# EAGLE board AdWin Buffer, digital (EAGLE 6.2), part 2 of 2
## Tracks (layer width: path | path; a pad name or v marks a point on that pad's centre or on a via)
+5V  (via drill 0.71)
  Top 0.406: IC3.21 301.75,53.75 301,53 301,49.25 299.5,47.75 298.5,47.75 C20.2 298.25,47.5 298,47.5 296.12,45.62 | 295.75,39.25 300.5,39.25 302.25,37.5 302.25,37 IC11.21 | 295.75,39.25 292,39.25 289.75,37 IC11.16 | 296.12,45.62 295.75,45.25 295.75,39.25 | 249.12,62.88 248.5,62.25 IC2.16 | 249.12,62.88 249.25,63 249.25,63.75 C4.2 | IC7.16 248.5,43 248.75,43.25 248.75,45.5 C18.2 249,45.75 249,46.75 250.12,47.88 | 250.62,61.38 250.75,61.25 250.75,48.5 250.12,47.88 | 250.62,61.38 249.12,62.88 | IC9.16 270.5,43.25 271.75,44.5 271.75,45.5 C16.2 271.75,45.75 271.75,47.5 | C5.2 271,64.5 271,62.25 270.75,62 IC1.16 | C3.2 287.5,65 287.5,66 286,67.5 283.25,67.5 282.25,66.5 273.75,66.5 272,64.75 271.38,64.75 C5.2 | 271.25,64.5 C5.2 | IC3.16 288.75,53.75 288.75,52.5 287.75,51.5 279.75,51.5 279.5,51.75 279.5,52.25 278.25,53.5 276.75,53.5 275.25,55 275.25,56.5 273.75,58 273.75,60.75 272.25,62.25 270.66,62.25 IC1.16 | 271.75,47.5 271.75,49.5 267.75,53.5 267.75,60.75 267.88,60.88 | 267.88,60.88 269.25,62.25 270.5,62.25 IC1.16 | 267.88,60.88 263.75,65 257.5,65 254,61.5 250.75,61.5 250.62,61.38 | 296.12,45.62 294.25,47.5 271.75,47.5 | F2.1A 182,59.75 172.5,69.25 167.75,69.25 C6.2 167.5,69.25 164,69.25 ZD1.2 163.75,69.25 163.25,68.75 161,68.75 159.48,67.23 147.51,67.23 143.25,62.75 142,62.75 141.75,63 120.75,63 v120.5,62.75 | C21.2 72.5,19.75 76.75,19.75 85.5,28.5 85.5,33.5 IC10.16 85.75,33.75 87,33.75 88,34.75 88,49.25 87.5,49.75 87.5,52 87.62,52.12 | 107.88,32.38 109,33.5 IC8.16 | 107.88,32.38 107,31.5 104.75,31.5 C19.2 | 104.75,40.75 104.75,35.5 107.88,32.38 | 104.75,40.75 104.75,41.25 C17.2
  Top 0.406: 104.75,40.75 106.5,42.5 v106.5,47.5 106.5,50 107.75,51.25 108.5,51.25 C10.2 108.75,51.5 108.75,53.25 109,53.5 IC4.16 109.25,53.25 v111,53.25 | 67.25,61.75 67.25,61 IC6.16 67.25,62 | IC6.21 54.75,61 61,67.25 61.5,67.25 C11.2 61.75,67.25 61.75,66.5 62.5,65.75 62.5,63.75 63.25,63 65.75,63 66.75,62 67.25,62 | 79.75,51.25 75.75,51.25 68.88,44.38 | 79.75,51.25 84.5,51.25 C9.2 84.75,51.5 84.75,52.5 85.5,53.25 IC5.16 85.75,53.25 86.5,53.25 87.62,52.12 | 68.88,44.38 67.5,43 67.5,42 IC12.16 | IC12.21 54.75,42 57.25,44.5 68.75,44.5 68.88,44.38 | 67.25,62 68.25,63 72.75,63 73.5,62.25 73.5,59.5 76,57 79,57 79.75,56.25 79.75,51.25 | 87.62,52.12 v92.25,47.5 | v243.75,50.25 244,50 248,50 250.12,47.88
  Bottom 0.406: v92.25,47.5 v106.5,47.5 | v111,53.25 v120.5,62.75 | F2.1A 182.25,59.5 216.25,59.5 222.5,53.25 240.75,53.25 v243.75,50.25
AGND  (via drill 0.71)
  other vias: 82.5,52.75 86.5,47.25 86.25,51.5 83.75,44.5 82.25,39 268.25,65.75 291.75,66.5 304,49 268.25,34.25 273.75,46 113.5,30.25 113.5,36.25 113.5,33.25 61.75,69 68.75,30.75 269,46 269,50.75 273.75,50.75 285.75,66.25 268.75,60.25 300.75,66.75 303.75,67
  pour Top (isolate 0.203): 0,96.52 0,5.08 169.03,5.08 169.03,0 330.2,0 330.2,96.52 171.45,96.52 171.45,88.9 164.47,88.9 164.47,92.08 158.12,92.08 158.12,96.52
  pour Bottom (isolate 0.203): 0,96.52 0,0 330.2,0 330.2,96.52
D0  (via drill 0.51)
  Top 0.178: v161.75,71 v165.25,71 | v139.75,55 138.5,53.75 138.5,49.75 J1.19 | IC2.3 239.25,59.75 239,59.5 237,59.5 236.75,59.25 v236.5,59.25
  Bottom 0.178: v165.25,71 170.75,65.5 222,65.5 228.25,59.25 v236.5,59.25 | v161.75,71 157.75,67 141.25,67 140,65.75 140,55.25 v139.75,55
D1  (via drill 0.51)
  Top 0.178: v156.75,64.5 167.75,64.5 176,56.25 226,56.25 235,65.25 240,65.25 243,62.25 243,60 241.5,58.5 239.5,58.5 IC2.4 | v139.75,53.75 139.75,47 J1.37
  Bottom 0.178: v156.75,64.5 156.25,64.5 154.25,66.5 141.5,66.5 140.5,65.5 140.5,54.5 v139.75,53.75
D2  (via drill 0.51)
  Top 0.178: v237.25,57.25 239.25,57.25 IC2.5 | v141,53.75 141,49.75 J1.18
  Bottom 0.178: v237.25,57.25 228.75,57.25 222.5,63.5 174.5,63.5 170.25,59.25 170.25,56.75 169.5,56 161.5,56 156.25,61.25 156.25,63.75 154,66 141.75,66 141,65.25 v141,53.75
D3  (via drill 0.51)
  Top 0.178: v237.25,56 239.25,56 IC2.6 | v165,53.25 162,53.25 159,50.25 159,49 158.25,48.25 154.5,48.25 153.5,49.25 153.5,50.25 152.25,51.5 146.5,51.5 145.25,50.25 145.25,49.25 143,47 142.5,47 J1.36
  Bottom 0.178: v237.25,56 229.25,56 222.25,63 174.75,63 170.75,59 170.75,56.62 168.5,54.38 166.25,54.38 165.12,53.25 v165,53.25
D4  (via drill 0.51)
  Top 0.178: v259.5,59.75 261.25,59.75 IC1.3 | v168.25,75 153.75,75 v143.5,64.75 | v143.25,56 143.25,50.25 143.75,49.75 J1.17
  Bottom 0.178: v259.5,59.75 248.25,59.75 240,68 181.25,68 174.25,75 v168.25,75 | v143.5,64.75 142.5,64.75 142,64.25 142,57.25 v143.25,56
D5  (via drill 0.51)
  Top 0.178: v263.25,58.5 261.5,58.5 IC1.4 | v163,63.75 156,63.75 v155.5,63.25
  Bottom 0.178: v263.25,58.5 262.75,58.5 260,55.75 250,55.75 247.5,58.25 228.5,58.25 222.75,64 163.25,64 v163,63.75 | v155.5,63.25 146.75,63.25 144.5,65.5 142,65.5 141.5,65 141.5,56.5 144.5,53.5 147.5,53.5 150.75,50.25 150.75,49.25 149.75,48.25 147,48.25 145.75,47 145.25,47 J1.35
D6  (via drill 0.51)
  Top 0.178: v259.5,57.75 260,57.25 261.25,57.25 IC1.5 | v177,67.5 168.75,75.75 v156.25,75.75 | v139,56.5 139.5,56.5 142.5,53.5 v142.5,52.25
  Bottom 0.178: v259.5,57.75 249.5,57.75 239.75,67.5 v177,67.5 | v156.25,75.75 148,67.5 141,67.5 139.5,66 139.5,57.25 139,56.75 v139,56.5 | v142.5,52.25 143.75,52.25 146.5,49.5 J1.16
D7  (via drill 0.51)
  Top 0.178: v259.5,56.5 260,56 261.25,56 IC1.6 | v230.5,65.25 182.75,65.25 169.5,78.5 150.25,78.5 v141,69.25 | v136.25,56.5 136.25,48 138.75,45.5 147,45.5 148.25,46.75 J1.34
  Bottom 0.178: v259.5,56.5 250,56.5 241.25,65.25 v230.5,65.25 | v141,69.25 138.25,66.5 138.25,58.5 v136.25,56.5
D8  (via drill 0.51)
  Top 0.178: v93,56 94.5,56 IC5.3
  Bottom 0.178: v93,56 97.75,51.25 128.5,51.25 130.25,53 145.75,53 149.25,49.5 J1.15
D9  (via drill 0.51)
  Top 0.178: v93,57.25 94.5,57.25 IC5.4
  Bottom 0.178: v93,57.25 92.25,56.5 92.25,55.5 97,50.75 122.5,50.75 129.5,43.75 148,43.75 151,46.75 J1.33
D10  (via drill 0.51)
  Top 0.178: v91.75,57.25 92.75,58.25 94.5,58.25 IC5.5 | J1.14 152.25,49.5 152.25,46.25 149.25,43.25 128.5,43.25 127.75,44 v127.75,44.25
  Bottom 0.178: v91.75,57.25 91.75,55.25 96.75,50.25 121.75,50.25 v127.75,44.25
D11  (via drill 0.51)
  Top 0.178: v91,55.25 91,57.75 92.75,59.5 94.5,59.5 IC5.6
  Bottom 0.178: v91,55.25 96.5,49.75 121,49.75 127.5,43.25 150.25,43.25 153.75,46.75 J1.32
D12  (via drill 0.51)
  Top 0.178: v116.5,56 118,56 IC4.3 | v125.5,57.25 147.25,57.25 154.75,49.75 J1.13
  Bottom 0.178: v116.5,56 124.25,56 v125.5,57.25
D13  (via drill 0.51)
  Top 0.178: v116.5,57.25 118,57.25 IC4.4 | v124.25,57.25 125,58 v145.75,58
  Bottom 0.178: v124.25,57.25 v116.5,57.25 | v145.75,58 153.5,50.25 153.5,49.25 155.75,47 156.25,47 J1.31
D14  (via drill 0.51)
  Top 0.178: v116,59.5 117,58.5 118,58.5 IC4.5 | v133.75,59 148,59 157.5,49.5 J1.12
  Bottom 0.178: v116,59.5 120.25,63.75 131,63.75 133.75,61 v133.75,59
D15  (via drill 0.51)
  Top 0.178: v142.75,63.75 118,63.75 116.5,62.25 116.5,60.25 117,59.75 118,59.75 IC4.6
  Bottom 0.178: v142.75,63.75 156.25,50.25 156.25,49.25 158.5,47 159,47 J1.30
D16  (via drill 0.51)
  Top 0.178: v255,39 255.25,38.75 262.75,38.75 263,39 263,39.75 262.25,40.5 261.5,40.5 IC9.3 | v246.5,31 179,31 165.25,44.75 162.75,44.75 v162.5,45
  Bottom 0.178: v255,39 254.5,39 v246.5,31 | v162.5,45 161.75,45 160.5,46.25 160.5,49.5 J1.11
D17  (via drill 0.51)
  Top 0.178: v167.5,48.5 168.75,47.25 168.75,46.25 182.75,32.25 241.75,32.25 244.5,35 244.5,38.5 247.25,41.25 259.5,41.25 259.75,41 259.75,40 260.25,39.5 261.25,39.5 IC9.4
  Bottom 0.178: v167.5,48.5 166.75,48.5 166.5,48.25 163.5,48.25 162,46.75 J1.29
D18  (via drill 0.51)
  Top 0.178: v166.75,53 163.25,49.5 J1.10 | IC9.5 261.34,38.25 254.5,38.25 253,39.75 v250.25,39.75
  Bottom 0.178: v250.25,39.75 246.25,39.75 244.25,41.75 218.25,41.75 212.25,47.75 212.25,51 210.25,53 v166.75,53
D19  (via drill 0.51)
  Top 0.178: v253.75,36.75 261.25,36.75 IC9.6 | v248.75,31.75 179.25,31.75 164.75,46.25 164.75,46.75 J1.28
  Bottom 0.178: v248.75,31.75 v253.75,36.75
D20  (via drill 0.51)
  Top 0.178: v241,40.5 239.5,40.5 IC7.3 | v176.25,36 166,46.25 166,49.5 J1.9
  Bottom 0.178: v241,40.5 241.75,39.75 241.75,36.25 241.5,36 v176.25,36
D21  (via drill 0.51)
  Top 0.178: v241,39.25 239.5,39.25 IC7.4 | v174.5,39.25 167.5,46.25 167.5,46.75 J1.27
  Bottom 0.178: v174.5,39.25 v241,39.25
D22  (via drill 0.51)
  Top 0.178: v241,38 239.5,38 IC7.5 | v179.75,38 171.5,46.25 171.5,47.25 169.25,49.5 168.75,49.5 J1.8
  Bottom 0.178: v179.75,38 v241,38
D23  (via drill 0.51)
  Top 0.178: v241,36.75 239.5,36.75 IC7.6 | v179.75,36.75 170.25,46.25 170.25,46.75 J1.26
  Bottom 0.178: v179.75,36.75 v241,36.75
D24  (via drill 0.51)
  Top 0.178: v93,36.25 94.5,36.25 IC10.3 | J1.7 171.25,49.5 169.25,51.5 166,51.5 164.5,50 164.5,49 163.75,48.25 161.25,48.25 160.5,47.5 160.5,46.5 156,42 126,42 124.5,43.5 v123.5,43.5
  Bottom 0.178: v93,36.25 98.25,36.25 104.75,42.75 122.75,42.75 v123.5,43.5
D25  (via drill 0.51)
  Top 0.178: v93,37.5 94.5,37.5 IC10.4 | v123.5,42.25 v122.25,43.5
  Bottom 0.178: v93,37.5 98.75,37.5 104.75,43.5 v122.25,43.5 | v123.5,42.25 163.25,42.25 166.5,45.5 171.25,45.5 172.75,47 J1.25
D26  (via drill 0.51)
  Top 0.178: v93,38.75 94.5,38.75 IC10.5 | v155,59.75 154.75,59.75 154.5,59.5 134.75,59.5 134.25,60 131.25,60 129.75,58.5 124.25,58.5 123.25,57.5 123.25,49.5 121.25,47.5 v121.25,47.25
  Bottom 0.178: v93,38.75 99.25,38.75 105.75,45.25 119.25,45.25 v121.25,47.25 | v155,59.75 163.25,51.5 172.25,51.5 174.25,49.5 J1.6
D27  (via drill 0.51)
  Top 0.178: v93,40 94.5,40 IC10.6 | v101.25,42 103.75,39.5 v103.75,39.25 | v176.25,42.75 176.25,46.25 175.75,46.75 J1.24
  Bottom 0.178: v93,40 99.25,40 v101.25,42 | v103.75,39.25 114.25,39.25 129.75,23.75 132.5,23.75 133.5,24.75 133.5,26.5 143.25,36.25 169.75,36.25 v176.25,42.75
D28  (via drill 0.51)
  Top 0.178: v117.75,44.5 116.5,43.25 116.5,36.75 117,36.25 118,36.25 IC8.3 | J1.5 176.75,49.5 171.25,55 161,55 155.5,60.5 154.25,60.5 153.75,60 137.5,60 v137,60.5 | v121,44.5 126.5,50 126.5,51.5 131.5,56.5 v133,56.5
  Bottom 0.178: v121,44.5 v117.75,44.5 | v137,60.5 v133,56.5
D29  (via drill 0.51)
  Top 0.178: v120,37.5 118.25,37.5 IC8.4
  Bottom 0.178: v120,37.5 160,37.5 167,44.5 176.25,44.5 178.5,46.75 J1.23
D30  (via drill 0.51)
  Top 0.178: v120,38.75 118.25,38.75 IC8.5
  Bottom 0.178: v120,38.75 160.5,38.75 166.75,45 175.75,45 177,46.25 177,47.25 179.25,49.5 179.75,49.5 J1.4
D31  (via drill 0.51)
  Top 0.178: v120,40 IC8.6 | v178.25,43.5 181,46.25 181,46.75 J1.22
  Bottom 0.178: v120,40 119.25,39.25 119.25,37 119.5,36.75 169,36.75 175.75,43.5 v178.25,43.5
N$1  (via drill 0.51)
  Top 0.178: v245.5,53 245.5,58 247,59.5 248.25,59.5 IC2.14 | v302,48.75 306.5,53.25 306.5,53.75 IC3.23
  Bottom 0.178: v245.5,53 249.75,48.75 v302,48.75
N$2  (via drill 0.51)
  Top 0.178: v246.75,53 246,53.75 246,57.25 247,58.25 248.25,58.25 IC2.13 | v302,50.25 304.25,52.5 304.25,53.75 IC3.22
  Bottom 0.178: v246.75,53 250.5,49.25 301,49.25 v302,50.25
N$3  (via drill 0.51)
  Top 0.178: v249.75,52.25 250.25,52.75 250.25,56.5 249.75,57 248.5,57 IC2.12
  Bottom 0.178: v249.75,52.25 273.5,52.25 276,49.75 295,49.75 299,53.75 IC3.20
N$4  (via drill 0.51)
  Top 0.178: v246.75,55.75 248.25,55.75 IC2.11
  Bottom 0.178: v246.75,55.75 249.25,55.75 249.75,55.25 271.25,55.25 276.25,50.25 293,50.25 296.5,53.75 IC3.19
N$5  (via drill 0.51)
  Top 0.178: v70.75,68 70,68.75 69.5,68.75 59.5,78.75 v59.5,79.25 | IC5.14 82.62,55.88 v77.25,61.25
  Bottom 0.178: v70.75,68 77.25,61.5 v77.25,61.25 | v59.5,79.25 51.5,79.25 49.25,77 49.25,61.25 49.5,61 IC6.23
N$6
  Top 0.178: IC5.13 85.75,57.25 86.75,57.25 88,58.5 88,63 83.75,67.25 66.25,67.25 63,70.5 60.5,70.5 52.25,62.25 52.25,61 IC6.22
N$7  (via drill 0.51)
  Top 0.178: v273.25,55.75 270.75,55.75 IC1.11
  Bottom 0.178: v273.25,55.75 276,55.75 279.5,52.25 282.25,52.25 283.75,53.75 IC3.14
N$8  (via drill 0.51)
  Top 0.178: v61.25,65.25 57,61 IC6.20 | IC5.12 85.75,58.5 86.75,58.5 87.5,59.25 87.5,62.75 84.5,65.75 65.25,65.75 64.75,65.25 v64.5,65.25
  Bottom 0.178: v61.25,65.25 v64.5,65.25
N$9  (via drill 0.51)
  Top 0.178: v66.5,64.25 77.75,64.25 82.25,59.75 85.5,59.75 IC5.11
  Bottom 0.178: v66.5,64.25 62.5,64.25 59.75,61.5 59.75,61 IC6.19
N$10  (via drill 0.51)
  Top 0.178: v286.75,56.5 281.5,56.5 281,56 v279.25,56 277.5,56 276.75,56.75 276.75,57.75 277,58 278,58 278.75,57.25 280.75,57.25 281,57.5 281,58.5 279,60.5 v279,63.5 | v295.75,66 296.5,65.25 296.5,61.75 IC3.6 | v279,68.5 287,68.5 v287.5,68
  Bottom 0.178: v279.25,56 280,56.75 283.25,56.75 R1.4A | v286.75,56.5 287.5,56.5 287.75,56.75 288.75,56.75 R2.4A | v295.75,66 294.5,66 292.5,68 v287.5,68 | v279,63.5 v279,68.5
N$11  (via drill 0.51)
  Top 0.178: v279.75,61 282.25,58.5 287.5,58.5 288,58 v293.5,58 | v288.25,56 v292.5,56 | v293,60 293.25,59.75 294.25,59.75 295,60.5 295,66.5 295.25,66.75 297.5,66.75 301.5,62.75 301.5,61.75 IC3.4
  Bottom 0.178: v279.75,61 278.25,59.5 278.25,55.75 278.75,55.25 279.75,55.25 280.75,56.25 281.75,56.25 282.25,55.75 283.25,55.75 284,56.5 284,56.75 R1.3A | v292.5,56 293.5,57 v293.5,58 293,58.5 v293,60 | v288.25,56 289.25,56 290,56.75 R2.3A
N$12  (via drill 0.51)
  Top 0.178: v277,51.5 278,50.5 289.75,50.5 v290.75,51.5 291.25,51 v297.5,51 | v309,51 310.75,52.75 310.75,56.25 309.5,57.5 308.6,57.5 306.85,59.25 305.75,59.25 304.25,60.75 304.25,61.54 IC3.3
  Bottom 0.178: v277,51.5 277.75,52.25 278.75,52.25 279.25,51.75 283.75,51.75 285,53 285,56.75 R1.2A | v290.75,51.5 290.75,51.75 290.5,52 290.5,56.75 R2.2A | v297.5,51 v309,51
N$13  (via drill 0.51)
  Top 0.178: v287.5,52.5 287.5,56.5 288.25,57.25 v292.5,57.25 293,57.25 295,55.25 295,53 296.25,51.75 v298.5,51.75
  Bottom 0.178: v287.5,52.5 287.5,55 286.75,55.75 286.25,55.75 285.75,56.25 285.75,56.75 R1.1A | v292.5,57.25 291.5,57.25 291.25,57 R2.1A | v298.5,51.75 310.75,51.75 311.75,52.75 311.75,60.25 311,61 309.87,61 IC3.1
N$14  (via drill 0.51)
  Top 0.178: v301,64.5 300.5,64.5 297.75,67.25 295,67.25 294.25,66.5 294.25,61.75 IC3.7 | v304.25,63.75 305.25,62.75 305.25,61 306.5,59.75 307.5,59.75 v309,58.25
  Bottom 0.178: v301,64.5 301.75,63.75 | 301.75,63.75 302.75,62.75 302.75,60.5 301.75,59.5 301.75,57.75 301,57 R4.1A | v309,58.25 307.75,57 306.75,57 R3.1A | 301.75,63.75 v304.25,63.75
N$15  (via drill 0.51)
  Top 0.178: IC3.9 288.75,61.5 291,59.25 294.25,59.25 295,58.5 298.25,58.5 300.25,56.5 302.75,56.5 | v307.5,56 306.25,56 305.75,56.5 302.75,56.5 | v302.75,57.5 302.75,56.5
  Bottom 0.178: v302.75,57.5 301.25,56 300.5,56 300.25,56.25 300.25,56.75 R4.2A | v307.5,56 307.25,55.75 306.5,55.75 306,56.25 306,56.75 R3.2A
N$16  (via drill 0.51)
  Top 0.178: v278.25,51.5 277.25,52.5 276.25,52.5 274.25,54.5 274.25,56 273.1,57.15 IC1.12
  Bottom 0.178: v278.25,51.5 278.75,51.5 279,51.25 284.25,51.25 286.25,53.25 286.25,53.75 IC3.15
N$17
  Top 0.178: IC3.17 291.25,53.75 291.25,53.25 289,51 279.25,51 279,51.25 279,52 278,53 276.5,53 274.75,54.75 274.75,56.25 273.25,57.75 272.25,57.75 271.58,58.42 IC1.13
N$18  (via drill 0.51)
  Top 0.178: v272.5,59.5 270.75,59.5 IC1.14
  Bottom 0.178: v272.5,59.5 272.5,54.75 276.5,50.75 291.25,50.75 294.25,53.75 IC3.18
N$19  (via drill 0.51)
  Top 0.178: 295.25,58 v297.5,55.75 | 295.25,58 294.75,58 294,58.75 288,58.75 287,59.75 287,61.01 IC3.10 | 295.25,58 298,58 300.25,55.75 v305.25,55.75
  Bottom 0.178: v297.5,55.75 298.5,55.75 299.25,56.5 299.25,56.75 R4.3A | v305.25,55.75 305.25,56.75 R3.3A
N$20  (via drill 0.51)
  Top 0.178: v308,52.5 308,55.25 308.25,55.5 308.25,56.4 307.9,56.75 306.25,56.75 304.75,58.25 301.5,58.25 300.75,57.5 300,57.5 298.25,59.25 v297.25,59.25
  Bottom 0.178: 295.75,57.75 295,58.5 295,63.25 293.25,65 287,65 286.25,64.25 283.5,64.25 281.5,62.25 281.5,61.75 IC3.12 | 295.75,57.75 297,56.5 298,56.5 298.25,56.75 298.5,56.75 R4.4A | R3.4A 303,55.75 303,53 303.75,52.25 307.75,52.25 v308,52.5 | 295.75,57.75 v297.25,59.25
N$21  (via drill 0.51)
  Top 0.178: v97.75,59.75 109,59.75 IC4.11
  Bottom 0.178: v97.75,59.75 83.75,59.75 79.25,55.25 78,55.25 72.75,60.5 72.75,60.6 IC6.14
N$22  (via drill 0.51)
  Top 0.178: v97.75,58.5 109,58.5 IC4.12 | v72.25,58.75 70,61 IC6.15
  Bottom 0.178: v72.25,58.75 73.5,58.75 77.5,54.75 79.5,54.75 84,59.25 96.75,59.25 97.5,58.5 v97.75,58.5
N$23  (via drill 0.51)
  Top 0.178: v97.75,57.25 109,57.25 IC4.13 | v78,54 77,54 73,58 68.25,58 67.5,58.75 66.5,58.75 65,60.25 65,60.75 IC6.17
  Bottom 0.178: v97.75,57.25 97.5,57.25 96,58.75 84.25,58.75 79.5,54 v78,54
N$24  (via drill 0.51)
  Top 0.178: v292.5,63.5 292.5,65.5 293,66 293,67.25 297.25,71.5 v298.5,71.5
  Bottom 0.178: v292.5,63.5 292.25,63.75 291.5,63.75 290.5,62.75 290.5,60.5 291.25,59.75 291.25,58.75 R2.1B | v298.5,71.5 299.5,71.5 315.5,87.5 319,87.5 D1.A
N$25  (via drill 0.51)
  Top 0.178: v97.75,48.5 105,55.75 109,55.75 IC4.14
  Bottom 0.178: v97.75,48.5 74.5,48.5 74,48 67.25,48 63.25,52 63.25,55.25 61.75,56.75 61.75,60.5 62,60.75 IC6.18
N$26  (via drill 0.51)
  Top 0.178: v53.5,51.75 54.25,51 57.75,51 59.5,52.75 59.5,53.25 IC6.6
  Bottom 0.178: R6.4A 48.25,55 48.25,51.75 49.5,50.5 57.25,50.5 59.5,52.75 59.5,53.25 IC6.6 | v53.5,51.75 53.5,55.25 54.5,56.25 R5.4A
N$27  (via drill 0.51)
  Top 0.178: v286.75,57.75 282,57.75 281,56.75 278,56.75 v277.5,57.25
  Bottom 0.178: v286.75,57.75 287.5,58.5 288.75,58.5 R2.4B | v277.5,57.25 277.5,73.5 273,78 263.75,78 258.25,83.5 258.25,87.5 D4.A
N$28  (via drill 0.51)
  Top 0.178: v288,72.25 288,69.25 289,68.25 289,64.5 287.75,63.25 287.75,60.25 v288.25,59.75
  Bottom 0.178: v288,72.25 288,74.75 283.25,79.5 283,79.5 278.5,84 278.5,87.5 D3.A | R2.3B 289.75,58.75 289.75,59.25 289.25,59.75 v288.25,59.75
N$29  (via drill 0.51)
  Top 0.178: v290,63.75 290,67.25 294,71.25 v294,76.25
  Bottom 0.178: v290,63.75 290,60.25 290.5,59.75 290.5,58.75 R2.2B | v294,76.25 298.5,80.75 298.5,87.5 D2.A
N$30
  Bottom 0.178: R6.3A 50.5,56.25 50.5,52.75 52.25,51 54,51 54.5,51.5 54.5,53.25 IC6.4 54.5,53.5 55.25,54.25 55.25,56.25 R5.3A
N$31  (via drill 0.51)
  Top 0.178: v55.75,51.75 55.75,54.5 54.75,55.5 53.75,55.5 52.25,54 52.25,53.5 IC6.3
  Bottom 0.178: R6.2A 51.25,56.25 51.25,55 52,54.25 52,53.5 IC6.3 | v55.75,51.75 55.75,54.25 56.25,54.75 56.25,56.25 R5.2A
N$32  (via drill 0.51)
  Top 0.178: IC6.1 47,53.5 47,54 49.25,56.25 v53,56.25 55.25,56.25 56,55.5 v58,55.5
  Bottom 0.178: v53,56.25 52,56.25 R6.1A | v58,55.5 57.25,56.25 R5.1A
N$33  (via drill 0.51)
  Top 0.178: IC6.7 62,53.5 64.75,56.25 v67,56.25 v72,56.25
  Bottom 0.178: v67,56.25 66,56.25 R7.1A | v72,56.25 71.25,56.25 R8.1A
N$34  (via drill 0.51)
  Top 0.178: v71,51.75 70.5,51.25 69,51.25 67.5,52.75 67.5,53.25 IC6.9
  Bottom 0.178: R7.2A 65.25,56.25 65.25,55.75 67.5,53.5 IC6.9 | R8.2A 70.25,55.25 71,54.5 v71,51.75
N$35  (via drill 0.51)
  Top 0.178: v67.25,50.75 72,50.75 73.75,52.5 73.75,54.75 73,55.5 71.25,55.5 70,54.25 70,53.5 IC6.10
  Bottom 0.178: v67.25,50.75 66.25,51.75 66.25,54 64.5,55.75 64.5,56.25 R7.3A | R8.3A 69.25,56.25 69.25,54 69.75,53.5 IC6.10
N$36
  Bottom 0.178: 68.75,51 67.75,50 66,50 63.75,52.25 63.75,56.25 R7.4A | 68.75,51 68.75,56.25 R8.4A | 68.75,51 73,51 74.75,52.75 74.75,53.25 IC6.12
N$37  (via drill 0.51)
  Top 0.178: v297.5,57.25 298,57.25 300.25,55 300.25,49.5 299.25,48.5 273.75,48.5 268.75,53.5 v268.75,56.25
  Bottom 0.178: v297.5,57.25 297.5,57.75 298.25,58.5 298.5,58.5 R4.4B | v268.75,56.25 256.5,68.5 201,68.5 184,85.5 179,85.5 177,87.5 D8.A
N$38  (via drill 0.51)
  Top 0.178: v56.75,68.5 50.5,62.25 50.5,60 51.75,58.75 v52.25,58.75 | v65,76 66.75,76 77,86.25 v149.25,86.25
  Bottom 0.178: v56.75,68.5 57.75,68.5 62.5,73.25 62.5,73.5 v65,76 | v149.25,86.25 150.5,87.5 151.25,87.5 D9.A | R6.1B 52,58.5 v52.25,58.75
N$39  (via drill 0.51)
  Top 0.178: v298,64 298,65 v297,66 | v199,86.75 v274.75,86.75 | v283.75,77.75 288.5,77.75 290.5,75.75 v290.5,71
  Bottom 0.178: v298,64 298,60.5 299.25,59.25 299.25,58.75 R4.3B | v290.5,71 294.75,66.75 296.25,66.75 v297,66 | v274.75,86.75 v283.75,77.75 | v199,86.75 198.25,87.5 197.25,87.5 D7.A
N$40  (via drill 0.51)
  Top 0.178: v219.5,86 278.5,86 279,86.5 283.25,86.5 292,77.75 295.75,77.75 301,72.5 301,70.5 302.75,68.75 302.75,60.5 302,59.75 v300,59.75
  Bottom 0.178: v300,59.75 300,58.75 R4.2B | v219.5,86 218,87.5 217.5,87.5 D6.A
N$41  (via drill 0.51)
  Top 0.178: v282.75,64.75 277.5,64.75 v276.5,63.75
  Bottom 0.178: v276.5,63.75 275,62.25 268.25,62.25 245,85.5 240,85.5 237.75,87.75 D5.A | R4.1B 300.75,58.75 300.75,60.25 300.5,60.5 300.5,63 298.75,64.75 294.25,64.75 293.5,65.5 286.75,65.5 286,64.75 v282.75,64.75
N$42  (via drill 0.51)
  Top 0.178: v77.5,85.5 v68.75,76.75
  Bottom 0.178: v68.75,76.75 56,76.75 51,71.75 51,58 R6.2B | v77.5,85.5 128.5,85.5 130.5,87.5 131,87.5 D10.A
N$43  (via drill 0.51)
  Top 0.178: v48.5,58.75 48.5,66.5 47,68 47,74.25 47.75,75 47.75,78.75 51.5,82.5 v51.5,83.5
  Bottom 0.178: v48.5,58.75 50,58.75 50.25,58.5 50.25,58 R6.3B | v51.5,83.5 52,83.5 54.5,86 63.25,86 67.5,90.25 108,90.25 110.5,87.75 D11.A
N$44  (via drill 0.51)
  Top 0.178: v45.5,76.25 v45.5,58.75
  Bottom 0.178: v45.5,58.75 46.25,58 49.5,58 R6.4B | v45.5,76.25 54.75,85.5 63.5,85.5 67.75,89.75 87.75,89.75 89.75,87.75 90.25,87.75 D12.A
N$45  (via drill 0.51)
  Top 0.178: v77,53.25 78.5,53.25 78.75,53.5 v78.75,56
  Bottom 0.178: v77,53.25 77,54.5 73.75,57.75 71.25,57.75 R8.1B | v78.75,56 78.75,64 72.5,70.25 72.5,73.25 75.25,76 75.25,77.5 70.25,82.5 70.25,87.5 D13.A
N$46  (via drill 0.51)
  Top 0.178: v69.5,68 57.75,79.75 57.75,83.75 55.75,85.75 v51.75,85.75
  Bottom 0.178: R8.2B 70.25,59.25 71,60 71,66.5 v69.5,68 | v51.75,85.75 50,87.5 D14.A
N$47  (via drill 0.51)
  Top 0.178: v68.25,68 68,68.25 68,68.75 57.25,79.5 57.25,83.5 55.75,85 51.25,85 v46.5,89.75
  Bottom 0.178: v68.25,68 68.75,67.5 68.75,59.75 69.25,59.25 69.25,58 R8.3B | v46.5,89.75 32,89.75 30,87.75 29.5,87.75 D15.A
N$48  (via drill 0.51)
  Top 0.178: v11.25,86 40,57.25 48,57.25 48.75,58 55.5,58 56.75,59.25 65,59.25 66.25,58 v67,58
  Bottom 0.178: v67,58 68.5,58 R8.4B | v11.25,86 9.75,87.5 9.25,87.5 D16.A
N$49
  Bottom 0.406: F2.2A 161.75,59.75 161.75,69.25 167,74.5 167,89.25 168.25,90.5 168.25,91.25 SUPPLY_+5V.P$1
N$50
  Top 0.203: 0,0.64 0,0 0.64,0
N$51
  Bottom 0.203: 0,0.64 0,0 0.64,0
N$52
  Top 0.203: 0.64,96.52 0,96.52 0,95.89
N$53
  Bottom 0.203: 0.64,96.52 0,96.52 0,95.89
N$54
  Top 0.203: 330.2,95.89 330.2,96.52 329.56,96.52
N$55
  Bottom 0.203: 330.2,95.89 330.2,96.52 329.56,96.52
N$56
  Top 0.203: 329.56,0 330.2,0 330.2,0.64
N$57
  Bottom 0.203: 329.56,0 330.2,0 330.2,0.64
N$58
  Top 0.406: J1.2 185.5,49.75 188.75,53 198,53 202.75,48.25 F1.1A
N$59  (via drill 0.51)
  Top 0.178: v274,34 274,39 272.5,40.5 270.75,40.5 IC9.14 | v295.75,28 300.25,28 v301,27.25
  Bottom 0.178: v274,34 274.5,34 280.5,28 v295.75,28 | v301,27.25 301,27.75 307.25,34 307.25,36.75 IC11.23
N$60  (via drill 0.51)
  Top 0.178: v272.5,39.25 270.75,39.25 IC9.13 | v298.25,30 v295.75,30
  Bottom 0.178: v272.5,39.25 281.75,30 v295.75,30 | v298.25,30 305,36.75 IC11.22
N$61  (via drill 0.51)
  Top 0.178: v272.5,38 270.75,38 IC9.12 | IC11.20 299.72,35.72 299,35 295.5,35 294.5,34 289.5,34 289,34.5 277,34.5 v276.5,34
  Bottom 0.178: v276.5,34 v272.5,38
N$62  (via drill 0.51)
  Top 0.178: v272.5,36.75 270.75,36.75 IC9.11 | v279.25,30.5 283,30.5 v284,31.5
  Bottom 0.178: v272.5,36.75 278.75,30.5 v279.25,30.5 | v284,31.5 292.75,31.5 297,35.75 297,36.75 IC11.19
N$63  (via drill 0.51)
  Top 0.178: v251,36.75 248.5,36.75 IC7.11 | v281,40.75 284.25,37.5 284.25,37 IC11.14
  Bottom 0.178: v251,36.75 251.5,36.75 256.75,42 279.75,42 v281,40.75
N$64
  Top 0.178: IC7.12 248.51,38 251.75,38 252.5,37.25 252.5,35 255.25,32.25 274.5,32.25 275.5,33.25 275.5,34.25 276.25,35 286,35 287.02,36.02 IC11.15
N$65  (via drill 0.51)
  Top 0.178: v299,29 v295,29 | v304.25,34.25 302.75,34.25 300.75,36.25 300.75,38 300,38.75 293.25,38.75 292.25,37.75 292.25,37 IC11.17 | IC7.13 248.25,39.25 246.25,39.25 245.5,38.5 245.5,32.75 245.75,32.5 250,32.5 252,30.5 276.5,30.5 278,32 v278,32.5
  Bottom 0.178: v278,32.5 278.5,32.5 282,29 v295,29 | v304.25,34.25 v299,29
N$66  (via drill 0.51)
  Top 0.178: v259,40.5 248.5,40.5 IC7.14 | v278,36.75 v273.5,41.25
  Bottom 0.178: v259,40.5 270.25,40.5 271,41.25 v273.5,41.25 | IC11.18 294.75,36.75 292,34 281.25,34 278.5,36.75 v278,36.75
N$67  (via drill 0.51)
  Top 0.178: IC11.6 297,44.25 299.75,41.5 v302.5,41.5 v308.25,41.5
  Bottom 0.178: v302.5,41.5 301.75,41.5 R9.4A | v308.25,41.5 307.5,41.5 R10.4A
N$68  (via drill 0.51)
  Top 0.178: v306.25,42.75 303.5,42.75 302.5,43.75 302.5,44.25 IC11.4
  Bottom 0.178: R9.3A 300.75,41.5 300.75,42 302.25,43.5 302.25,44.25 IC11.4 | v306.25,42.75 306.25,41.5 R10.3A
N$69
  Bottom 0.178: R9.2A 300,41.5 300,42 301.25,43.25 301.25,45.75 301.75,46.25 303.25,46.25 305,44.5 IC11.3 304.75,44.25 305.5,43.5 305.5,41.5 R10.2A
N$70  (via drill 0.51)
  Top 0.178: v303.5,40.75 308.75,40.75 309.75,41.75 309.75,44.25 IC11.1
  Bottom 0.178: R9.1A 299,41.5 299,42.25 298.25,43 298.25,45.75 299.75,47.25 307.5,47.25 309.75,45 309.75,44.5 IC11.1 | v303.5,40.75 304.25,41.25 304.75,41.25 R10.1A
N$71  (via drill 0.51)
  Top 0.178: v283.25,43 283.5,42.75 283.75,42.75 285.25,41.25 288.25,41.25 v288.5,41.5 288.75,41.25 292.25,41.25 294.64,43.64 IC11.7
  Bottom 0.178: v283.25,43 283.25,42.75 284.5,41.5 R11.1A | v288.5,41.5 289.5,41.5 R12.1A
N$72  (via drill 0.51)
  Top 0.178: v285.5,42.75 288.25,42.75 289.75,44.25 IC11.9
  Bottom 0.178: v285.5,42.75 285.5,41.5 R11.2A | R12.2A 290.25,41.5 290.25,43.5 289.5,44.25 IC11.9
N$73  (via drill 0.51)
  Top 0.178: v291,42.75 291,45.5 290.25,46.25 288.25,46.25 287.25,45.25 287.25,44.5 IC11.10
  Bottom 0.178: R11.3A 286.25,41.5 286.25,43.25 287.25,44.25 IC11.10 | v291,42.75 291,41.5 R12.3A
N$74
  Bottom 0.178: 287,46.75 288,45.75 288,42.5 287,41.5 R11.4A | 287,46.75 284,46.75 281.75,44.5 IC11.12 | 287,46.75 292.5,46.75 293.5,45.75 293.5,42.75 292.25,41.5 R12.4A
N$75  (via drill 0.51)
  Top 0.178: v304.5,39 310.5,39 v319,30.5
  Bottom 0.178: v304.5,39 304.75,39.75 R10.1B | v319,30.5 319,25.5 D17.A
N$76
  Bottom 0.178: R10.2B 305.75,39.75 305.75,38 306.25,37.5 306.25,33.75 298.75,26.25 298.75,25.5 D18.A
N$77  (via drill 0.51)
  Top 0.178: v280.5,26.75 283.5,26.75 290.25,33.5 294.75,33.5 295.75,34.5 301.75,34.5 302.75,33.5 308,33.5 v308.5,34
  Bottom 0.178: v308.5,34 308.5,37.75 307.75,38.5 307.25,38.5 306.5,39.25 306.5,39.75 R10.3B | v280.5,26.75 279.25,25.5 278.5,25.5 D19.A
N$78
  Bottom 0.178: R10.4B 307.5,39.75 309.75,39.75 311.5,38 311.5,21.5 303,13 286.25,13 271.75,27.5 260.75,27.5 258.75,25.5 258.25,25.5 D20.A
N$79  (via drill 0.51)
  Top 0.178: v288.25,38.5 288.25,36 289.5,34.75 v294,34.75 | v280,33.25 273.5,26.75 v239.75,26.75
  Bottom 0.178: v288.25,38.5 289.5,39.75 R12.1B | v294,34.75 293.5,34.75 292,33.25 v280,33.25 | v239.75,26.75 238.5,25.5 237.75,25.5 D21.A
N$80  (via drill 0.51)
  Top 0.178: v259.25,27.5 220.25,27.5 v219.5,26.75
  Bottom 0.178: v259.25,27.5 271.75,40 276,40 281.5,34.5 290,34.5 291,35.5 291,37.5 290.5,38 290.5,39.75 R12.2B | v219.5,26.75 218.25,25.5 217.5,25.5 D22.A
N$81  (via drill 0.51)
  Top 0.178: v247.5,47.25 247.5,47 242,41.5 242,36.25 v241,35.25
  Bottom 0.178: v247.5,47.25 294,47.25 295.75,45.5 295.75,42.25 292.5,39 291.5,39 291.25,39.25 291.25,39.75 R12.3B | v241,35.25 215.25,35.25 207.5,27.5 199.75,27.5 197.75,25.5 197.25,25.5 D23.A
N$82  (via drill 0.51)
  Top 0.178: v293,40.75 285,40.75 283.5,42.25 277.75,42.25 v275,45 | v210.5,34 v219,42.5
  Bottom 0.178: v293,40.75 292.25,40 R12.4B | v219,42.5 253.25,42.5 255.5,44.75 274.5,44.75 274.75,45 v275,45 | v210.5,34 185.75,34 177,25.25 D24.A
N$83  (via drill 0.51)
  Top 0.178: v83.25,47.5 87.5,43.25 87.5,37 86.75,36.25 85.75,36.25 IC10.14
  Bottom 0.178: v83.25,47.5 51.5,47.5 49.75,45.75 49.75,42 IC12.23
N$84  (via drill 0.51)
  Top 0.178: v72.5,46.75 83.25,46.75 87,43 87,38.25 86.25,37.5 85.75,37.5 IC10.13
  Bottom 0.178: v72.5,46.75 56,46.75 52.25,43 52.25,42 IC12.22
N$85  (via drill 0.51)
  Top 0.178: v83.75,38.75 85.5,38.75 IC10.12
  Bottom 0.178: v83.75,38.75 77.75,44.75 59.75,44.75 57,42 IC12.20
N$86  (via drill 0.51)
  Top 0.178: v81.25,40 85.5,40 IC10.11
  Bottom 0.178: v81.25,40 79.75,40 75.5,44.25 61.75,44.25 59.5,42 IC12.19
N$87  (via drill 0.51)
  Top 0.178: v105.75,40 109,40 IC8.11
  Bottom 0.178: v105.75,40 102.75,40 98.25,35.5 80.25,35.5 76,39.75 74.75,39.75 72.5,42 IC12.14
N$88  (via drill 0.51)
  Top 0.178: v105.75,38.5 109,38.5 IC8.12 | IC12.15 69.75,42 72,44.25 75,44.25 77,42.25 77,40.25 82.25,35 v82.25,34.75
  Bottom 0.178: v105.75,38.5 102,38.5 98.5,35 82.5,35 v82.25,34.75
N$89  (via drill 0.51)
  Top 0.178: v106.5,37.25 109,37.25 IC8.13 | v79.5,34 78.75,34.75 77.5,34.75 76.75,34 76.75,30.75 72.75,30.75 v71.75,31.75
  Bottom 0.178: v106.5,37.25 101.5,37.25 98.75,34.5 83.25,34.5 82.75,34 v79.5,34 | v71.75,31.75 64.75,31.75 63.25,33.25 63.25,36.5 63,36.75 63,39.25 64.75,41 64.75,41.75 IC12.17
N$90  (via drill 0.51)
  Top 0.178: v105.75,36.25 109,36.25 IC8.14 | v62.25,38 62.25,38.25 63.25,39.25 66.75,39.25 68.5,41 68.5,42.75 70.5,44.75 75.25,44.75 77.5,42.5 77.5,40.5 82.5,35.5 82.75,35.5 83.75,34.5 v83.75,33.75
  Bottom 0.178: v105.75,36.25 103,36.25 99.25,32.5 85,32.5 v83.75,33.75 | v62.25,38 62.25,41.75 IC12.18
N$91
  Bottom 0.178: 53.5,32 57.75,32 59.5,33.75 59.5,34.25 IC12.6 | 53.5,32 47,32 45.75,33.25 45.75,35.5 47.5,37.25 48.75,37.25 R14.4A | 53.5,32 53.5,35.25 54,35.75 54,37.25 R13.4A
N$92  (via drill 0.51)
  Top 0.178: v48.5,36 49,36.5 52.5,36.5 54.5,34.5 IC12.4
  Bottom 0.178: v48.5,36 49,36.5 49.5,36.5 49.75,36.75 49.75,37.25 R14.3A | R13.3A 54.75,37.25 54.75,34.5 IC12.4
N$93  (via drill 0.51)
  Top 0.178: v55.75,32.75 55.25,32.25 53.75,32.25 52.25,33.75 52.25,34.25 IC12.3
  Bottom 0.178: R14.2A 50.75,37.25 50.75,36.5 52,35.25 52,34.5 IC12.3 | v55.75,32.75 55.75,37.25 R13.2A
N$94  (via drill 0.51)
  Top 0.178: IC12.1 47,34.5 47,35.75 48.5,37.25 v52.5,37.25 v57.5,37.25
  Bottom 0.178: v52.5,37.25 51.5,37.25 R14.1A | v57.5,37.25 56.5,37.25 R13.1A
N$95  (via drill 0.51)
  Top 0.178: v68.5,38.75 73,38.75 v74,37.75
  Bottom 0.178: v68.5,38.75 67.25,37.5 R15.1A | R16.1A 73,37.5 73.75,37.5 v74,37.75 76.5,35.25 76.5,33.25 73,29.75 67.25,29.75 66.75,30.25 65.25,30.25 62.25,33.25 62.25,34.25 IC12.7
N$96  (via drill 0.51)
  Top 0.178: v71,32.75 70.25,32 69.25,32 67.5,33.75 67.5,34.25 IC12.9
  Bottom 0.178: R15.2A 66.5,37.25 66.5,35.5 67.5,34.5 IC12.9 | v71,32.75 71,35 72,36 72,37.25 R16.2A
N$97
  Bottom 0.178: R15.3A 65.75,37.25 65.75,33.75 67.25,32.25 68,32.25 70,34.25 IC12.10 70,34.5 70,35.5 71.25,36.75 71.25,37.25 R16.3A
N$98  (via drill 0.51)
  Top 0.178: v63.75,37.25 67,37.25 67.75,38 69.5,38 | 69.5,38 71.75,38 74.75,35 74.75,34.5 IC12.12 | 69.5,38 v69.5,37.25
  Bottom 0.178: v63.75,37.25 64.75,37.25 R15.4A | v69.5,37.25 70.5,37.25 R16.4A
N$99  (via drill 0.51)
  Top 0.178: v51,44.5 51,47 52.75,48.75 v70.75,48.75 | v88.5,50 88.5,39.25 91.75,36 v91.75,31.75
  Bottom 0.178: v51,44.5 51,40.75 51.25,40.5 51.25,39 R14.1B | v70.75,48.75 72,50 v88.5,50 | v91.75,31.75 121,31.75 129.5,23.25 148.75,23.25 150.75,25.25 151.25,25.25 D25.A
N$100  (via drill 0.51)
  Top 0.178: v52,46.75 70,46.75 v72,48.75 | v115,40.5 v109.5,46
  Bottom 0.178: v52,46.75 50.25,45 50.25,44 50.5,43.75 50.5,39 R14.2B | v72,48.75 74,48.75 74.5,49.25 106.25,49.25 v109.5,46 | v115,40.5 130,25.5 131,25.5 D26.A
N$101  (via drill 0.51)
  Top 0.178: v81,28.75 76.5,24.25 64.25,24.25 63.5,25 53,25 52.25,24.25 49,24.25 v45.5,27.75
  Bottom 0.178: v81,28.75 107,28.75 110.5,25.25 D27.A | R14.3B 49.75,39 49.75,39.5 49.5,39.75 46.75,39.75 42.75,35.75 42.75,30.5 v45.5,27.75
N$102  (via drill 0.51)
  Top 0.178: v65.5,28.75 v55.75,28.75 | v68,26.25 76.5,26.25 v76.75,26.5
  Bottom 0.178: v55.75,28.75 49.5,28.75 45.25,33 45.25,35.75 48.25,38.75 48.75,38.75 R14.4B | v68,26.25 v65.5,28.75 | v76.75,26.5 89.25,26.5 90.25,25.5 D28.A
N$103  (via drill 0.51)
  Top 0.178: v78,34 77.25,33.25 77.25,29.5 75.5,27.75 v71.25,27.75
  Bottom 0.178: v78,34 78,36.25 77.75,36.5 76.5,36.5 74.25,38.75 73,38.75 R16.1B | v71.25,27.75 70.25,26.75 70.25,25.5 D29.A
N$104  (via drill 0.51)
  Top 0.178: v51.75,25.5 64.75,25.5 66.25,27 75.5,27 78,29.5 v78,32.75
  Bottom 0.178: v78,32.75 78.75,33.5 78.75,36.25 78,37 76.75,37 73.75,40 72.75,40 72.25,39.5 72.25,39 R16.2B | v51.75,25.5 50,25.5 D30.A
N$105  (via drill 0.51)
  Top 0.178: v73.5,43.5 73.5,40.5 77.5,36.5 78.25,36.5 80.25,34.5 80.25,28.75 76.5,25 v66,25 | v61.5,20.5 54,13 42.25,13 v31.5,23.75
  Bottom 0.178: v73.5,43.5 73.25,43.75 72,43.75 71.25,43 71.25,39 R16.3B | v61.5,20.5 v66,25 | v31.5,23.75 30,25.25 29.5,25.25 D31.A
N$106  (via drill 0.51)
  Top 0.178: v68.25,37.25 67.75,37.25 66.25,35.75 66.25,33 v63.25,30 | v61.25,30 43.75,30 42.5,28.75 12.5,28.75 v9.25,25.5
  Bottom 0.178: v68.25,37.25 69.75,38.75 70.5,38.75 R16.4B | v61.25,30 v63.25,30 | 9.75,25.5 v9.25,25.5 D32.A
N$107  (via drill 0.51)
  Top 0.178: v44.75,25.75 45.25,25.75 47.25,23.75 52.5,23.75 53.25,24.5 61.25,24.5 62.75,23 62.75,17.75 74.5,6 143.5,6 152.25,14.75 BNC25.CONDUCTOR | v59,36.75 59,36.5 58.5,36 58.5,32.75 57,31.25 42,31.25 41.5,30.75 v40,30.75
  Bottom 0.178: R13.1B 56.5,38.75 58.25,38.75 59,38 v59,36.75 | v40,30.75 40,30.5 v44.75,25.75
N$108  (via drill 0.51)
  Top 0.178: v63.75,38.5 63,37.75 63,35.75 63.25,35.5 63.25,33 62,31.75 62,29.5 61.75,29.25 56.5,29.25 56.25,29.5 44,29.5 42.75,28.25 23.5,28.25 10,14.75 BNC32.CONDUCTOR
  Bottom 0.178: v63.75,38.5 64,38.75 64.75,38.75 R15.4B
N$109  (via drill 0.51)
  Top 0.178: v65.75,40.25 65.75,43 64.75,44 62.25,44 61.25,43 v61.25,39.5
  Bottom 0.178: v65.75,40.25 65.75,39 R15.3B | v61.25,39.5 61.25,33 55.75,27.5 48.25,27.5 33.75,13 31.75,13 30.25,14.5 BNC31.CONDUCTOR
N$110  (via drill 0.51)
  Top 0.178: v63.5,43.25 63.5,40.5 61.25,38.25 v61.25,31.25 | v58.75,23 51,15.25 51,14.75 BNC30.CONDUCTOR
  Bottom 0.178: v63.5,43.25 64,43.75 67.75,43.75 68.5,43 68.5,41 67.5,40 67,40 66.5,39.5 66.5,39 R15.2B | v61.25,31.25 58.75,28.75 v58.75,23
N$111  (via drill 0.51)
  Top 0.178: v69,40 69.25,39.75 73.25,39.75 v77.25,35.75
  Bottom 0.178: v69,40 68.25,40 67.25,39 R15.1B | v77.25,35.75 77.25,31.25 72.25,26.25 72.25,16 71,14.75 BNC29.CONDUCTOR
N$112  (via drill 0.51)
  Top 0.178: v55.75,40.25 55.5,40 54.25,40 53.5,40.75 53.5,43 v56.5,46 | v90.25,36.25 90.25,28.75 95.75,23.25 114.5,23.25 123,14.75 132,14.75 BNC26.CONDUCTOR
  Bottom 0.178: v55.75,40.25 55.75,39 R13.2B | v56.5,46 80.5,46 v90.25,36.25
N$113  (via drill 0.51)
  Top 0.178: v89,36.25 89,29.25 103.5,14.75 111.75,14.75 BNC27.CONDUCTOR
  Bottom 0.178: v89,36.25 80,45.25 55.75,45.25 53.5,43 53.5,40.75 54.75,39.5 54.75,39 R13.3B
N$114  (via drill 0.51)
  Top 0.178: v52.5,39.75 49.5,39.75 44,34.25 v44,32.5 | v48.75,28.25 50.25,26.75 55.75,26.75 56.25,26.25 v56.5,26.25
  Bottom 0.178: v52.5,39.75 53.25,39 54,39 R13.4B | v56.5,26.25 56.5,24 67.5,13 89.5,13 91.25,14.75 BNC28.CONDUCTOR | v48.75,28.25 44.5,32.5 v44,32.5
N$115  (via drill 0.51)
  Top 0.178: BNC17.CONDUCTOR 320,14.75 312,14.75 309,17.75 309,30 308,31 300.5,31 298.75,32.75 v296.5,32.75
  Bottom 0.178: v296.5,32.75 298.25,34.5 298.25,38.25 299,39 299,39.75 R9.1B
N$116
  Bottom 0.178: R9.2B 299.75,39.75 299.75,39 298.75,38 298.75,33.75 296.5,31.5 296.5,23 299.5,20 299.5,14.75 BNC18.CONDUCTOR
N$117  (via drill 0.51)
  Top 0.178: v297.75,31.5 294,31.5 279.5,17 279.5,14.71 BNC19.CONDUCTOR
  Bottom 0.178: v297.75,31.5 300.75,34.5 300.75,39.75 R9.3B
N$118  (via drill 0.51)
  Top 0.178: v302.25,39 301.5,39 300.25,40.25 v298,40.25 | v280.75,32.25 279.75,32.25 263.75,16.25 261,16.25 259.25,14.5 BNC20.CONDUCTOR
  Bottom 0.178: v302.25,39 301.75,39.75 R9.4B | v298,40.25 295.75,38 295.75,35.25 292.75,32.25 v280.75,32.25
N$119  (via drill 0.51)
  Top 0.178: v288,39.75 285.25,39.75 283.25,41.75 277.5,41.75 275.75,43.5 v273.25,43.5 | v241.75,28.75 192.25,28.75 178,14.5 BNC24.CONDUCTOR
  Bottom 0.178: v288,39.75 287,39.75 R11.4B | v241.75,28.75 256.5,43.5 v273.25,43.5
N$120  (via drill 0.51)
  Top 0.178: v286,38.5 285.25,38.5 v282.75,41
  Bottom 0.178: v286,38.5 286,39.75 R11.3B | v282.75,41 282,41 278.75,44.25 256,44.25 239.25,27.5 215.75,27.5 204.5,16.25 200,16.25 198.25,14.5 BNC23.CONDUCTOR
N$121  (via drill 0.51)
  Top 0.178: v278.25,39 277,39 274,42 272.5,42 271.75,41.25 269.25,41.25 v266.5,38.5
  Bottom 0.178: v278.25,39 285,39 285.25,39.25 285.25,39.75 R11.2B | BNC22.CONDUCTOR 218.25,14.5 219.75,13 221.75,13 232,23.25 243.5,23.25 256.75,36.5 264.5,36.5 v266.5,38.5
N$122
  Bottom 0.178: R11.1B 284.5,40 276.75,40 276.25,40.5 271,40.5 258,27.5 256.5,27.5 242,13 240.5,13 239,14.5 BNC21.CONDUCTOR
N$123  (via drill 0.51)
  Top 0.178: v286,59.5 283.75,59.5 282.75,60.5 282.75,63 v281.75,64 | v288.25,67 287.25,67 286.25,68 282.25,68 v281.75,67.5
  Bottom 0.178: v286,59.5 285.75,58.75 R1.1B | BNC1.CONDUCTOR 320,77 315.25,77 303.5,65.25 294.5,65.25 292.25,67.5 289,67.5 288.5,67 v288.25,67 | v281.75,67.5 v281.75,64
N$124  (via drill 0.51)
  Top 0.178: v73.25,75.25 89.5,75.25 91.25,77 BNC12.CONDUCTOR
  Bottom 0.178: v73.25,75.25 65,75.25 63,73.25 63,73 53.5,63.5 53.5,59 54.5,58 R5.4B
N$125  (via drill 0.51)
  Top 0.178: v55.5,59.25 54.25,59.25 53.5,60 53.5,62.75 60.75,70 62.75,70 66.25,66.5 v83.25,66.5
  Bottom 0.178: v55.5,59.25 55.5,58 R5.3B | v83.25,66.5 96.75,66.5 107.25,77 111.75,77 BNC11.CONDUCTOR
N$126  (via drill 0.51)
  Top 0.178: v68.5,74.5 74.75,68.25 123.25,68.25 132,77 BNC10.CONDUCTOR
  Bottom 0.178: v68.5,74.5 65,74.5 63.5,73 63.5,72.75 56,65.25 56,60 56.25,59.75 56.25,58 R5.2B
N$127  (via drill 0.51)
  Top 0.178: v70.5,71.25 74,67.75 143,67.75 152.25,77 BNC9.CONDUCTOR
  Bottom 0.178: v70.5,71.25 69.5,71.25 66.75,68.5 63.25,68.5 58.25,63.5 58.25,59 57.25,58 R5.1B
N$128  (via drill 0.51)
  Top 0.178: v68,55.25 67,55.25 66.25,54.5 66.25,52 64.25,50 v60.25,50 | v56.5,77.5 v48.5,69.5
  Bottom 0.178: v68,55.25 68,56.5 67.5,57 66.75,57 66,57.75 R7.1B | v60.25,50 46.75,50 44.75,52 44.75,65.75 v48.5,69.5 | v56.5,77.5 70.5,77.5 71,77 BNC13.CONDUCTOR
N$129  (via drill 0.51)
  Top 0.178: v62.5,57.25 62.5,55.75 61,54.25 61,52 60.5,51.5 59,51.5 58,50.5 41.5,50.5 13.5,78.5 11.5,78.5 10,77 BNC16.CONDUCTOR
  Bottom 0.178: v62.5,57.25 63,57.75 63.5,57.75 R7.4B
N$130
  Bottom 0.178: R7.3B 64.25,58 64.25,59.25 63.25,60.25 63.25,62.25 62.75,62.75 61.75,62.75 61.25,62.25 61.25,51.75 62.25,50.75 62.25,49.5 61.5,48.75 44,48.75 30.25,62.5 30.25,76.75 BNC15.CONDUCTOR
N$131  (via drill 0.51)
  Top 0.178: v69.75,70.25 68.75,70.25 61,78 v61,78.5
  Bottom 0.178: v69.75,70.25 69.25,70.25 67.5,68.5 67.5,64 65.75,62.25 65.75,59.75 65.25,59.25 65.25,58 R7.2B | v61,78.5 52.75,78.5 51,76.75 BNC14.CONDUCTOR
N$132  (via drill 0.51)
  Top 0.178: v285,63.25 284.25,64 v284.25,65.5
  Bottom 0.178: v285,63.25 285,58.75 R1.2B | BNC2.CONDUCTOR 299.5,76.75 297.5,74.75 293,74.75 290.5,72.25 290,72.25 284.25,66.5 v284.25,65.5
N$133  (via drill 0.51)
  Top 0.178: v274.5,63 v279,58.5 | v273.75,68 273.75,71.5 279.25,77 BNC3.CONDUCTOR
  Bottom 0.178: v279,58.5 280,59.5 283.75,59.5 284,59.25 284,58.75 R1.3B | v274.5,63 273.75,63.75 v273.75,68
N$134  (via drill 0.51)
  Top 0.178: v280.25,58 280.25,58.5 v274.5,64.25
  Bottom 0.178: v280.25,58 280.75,58.5 283.25,58.5 R1.4B | BNC4.CONDUCTOR 259.25,77 261,75.25 275,75.25 277,73.25 277,70.25 274.5,67.75 v274.5,64.25
N$135  (via drill 0.51)
  Top 0.178: v310.75,59 310.75,72.25 297.5,85.5 v288.5,85.5 | v279.25,85.5 247.75,85.5 239,76.75 BNC5.CONDUCTOR
  Bottom 0.178: v310.75,59 308,59 307.75,58.75 306.75,58.75 R3.1B | v279.25,85.5 v288.5,85.5
N$136  (via drill 0.51)
  Top 0.178: v312,69 312.75,69.75 312.75,73.75 297.5,89 v235.5,89
  Bottom 0.178: v312,69 307.75,64.75 307.75,60.5 307,59.75 306.5,59.75 306,59.25 306,58.75 R3.2B | v235.5,89 221.75,75.25 220.25,75.25 218.5,77 BNC6.CONDUCTOR
N$137  (via drill 0.51)
  Top 0.178: v312,70.25 312,73.75 297.5,88.25 v214.25,88.25
  Bottom 0.178: v312,70.25 305.75,64 305.75,60.25 305.25,59.75 305.25,58.75 R3.3B | v214.25,88.25 201.25,75.25 200,75.25 198.25,77 BNC7.CONDUCTOR
N$138  (via drill 0.51)
  Top 0.178: v305.25,65.75 305.25,67 301.5,70.75 301.5,72.75 296,78.25 292.25,78.25 283,87.5 188.75,87.5 178,76.75 BNC8.CONDUCTOR
  Bottom 0.178: v305.25,65.75 305.25,60.5 304.25,59.5 304.25,58.75 R3.4B
W+5V  (via drill 0.71)
  Top 0.406: 117.62,49.88 117.25,50.25 v117.25,52.25 117.25,52.5 118,53.25 IC4.1 | 117.62,49.88 118.5,49 C7.2 | 116.12,34.38 116,34.5 116,48.25 117.62,49.88 | 116.12,34.38 116.75,33.75 118,33.75 IC8.1 | IC5.1 94.5,53.25 93.75,52.5 93.75,49.5 94.25,49 95.25,49 C8.2 v95.25,44 | 94.75,32.25 94.75,33.5 IC10.1 | 94.75,32.25 94.75,31.25 C15.2 | 99.5,39.75 99.5,37 97.88,35.38 | 99.5,39.75 99.5,40 C13.2 99.5,39.75 | 94.75,32.25 97.88,35.38 | 99.5,39.75 v98.25,41 | 97.88,35.38 103.25,30 108,30 112.25,34.25 116,34.25 116.12,34.38 | IC9.1 261.5,43.25 261.5,45.5 C12.2 261.5,45.75 261,45.75 256.88,49.88 | IC1.1 261.25,62.25 260,63.5 C2.2 258,63.5 256.75,62.25 256.75,50 256.88,49.88 | IC2.1 239.25,62 238.5,62.75 236.25,62.75 C1.2 236,62.75 223.25,50 223.25,48.5 F1.2A 223,48.5 217,54.5 174.25,54.5 173.25,55.5 161.25,55.5 155.5,61.25 154,61.25 153.5,60.75 138.25,60.75 137.5,61.5 136.75,61.5 136,60.75 v130.75,60.75 | C14.2 239,45.5 v239,44.25 239,43.25 239.25,43 IC7.1 | v253,46 256.88,49.88
  Bottom 0.406: v98.25,41 v95.25,44 | F1.2A 223.25,48.25 227.25,44.25 v239,44.25 251.25,44.25 v253,46 | v117.25,52.25 125.25,52.25 130.75,57.75 v130.75,60.75
WGND  (via drill 0.71)
  Top 0.406: 121,38.75 121,41 119.5,42.5 118.25,42.5 IC8.8 118.25,42.75 118.25,43.75 118.75,44.25 118.75,46.75 120,48 120,50 119.25,50.75 118.8,50.75 C7.1 118.75,51 118.75,51.5 120.25,53 120.25,53.75 120.12,53.88 | 121,38.75 121,36.25 119.75,35 118.25,35 IC8.2 | 120.12,53.88 119.5,54.5 118.25,54.5 IC4.2 118,54.75 116.5,54.75 111,60.25 111,63 110.5,63.5 98.5,63.5 96.62,61.62 | IC4.8 118.25,62.25 119.5,62.25 120.25,61.5 120.25,54 120.12,53.88 | 96.62,53.88 96,54.5 94.75,54.5 IC5.2 | 96.62,53.88 96.75,53.75 96.75,53 95.25,51.5 C8.1 95.25,50.75 96.5,49.5 96.5,42.75 96.25,42.5 96,42.5 | 96.62,61.62 96.75,61.5 96.75,54 96.62,53.88 | 96.62,61.62 96,62.25 94.75,62.25 IC5.8 | 96.75,42 96.5,42 96,42.5 | 96.75,42 99.5,42 C13.1 | 96,42.5 94.75,42.5 IC10.8 | C15.1 94.5,29.25 94,29.25 93,30.25 93,34.25 93.75,35 94.5,35 IC10.2 94.75,35 96.25,35 96.75,35.5 96.75,42 | IC9.8 261.5,34.25 262.75,34.25 264.25,35.75 264.25,42 | 258.5,61.5 259.75,61.5 260.25,61 261.25,61 IC1.2 | 261.5,47.75 261.5,53.25 IC1.8 261.25,53.25 260.25,53.25 258.62,54.88 | 261.5,47.75 C12.1 | 258.5,61.5 258.5,55 258.62,54.88 | 258.5,61.5 C2.1 | J1.21 183.75,47 182.75,48 182.75,49.5 J1.3 | 237.88,41.88 238,42 239.25,42 IC7.2 | 237.88,41.88 237.25,41.25 237.25,35 238,34.25 239.25,34.25 IC7.8 | IC2.2 239.25,61 236.25,61 C1.1 236.25,60.75 235,60.75 233.75,59.5 233.75,53.75 234.16,53.34 IC2.8 | IC2.8 239.25,53.5 239,53.25 239,47.75 C14.1 238.75,47.5 237.75,47.5 237.25,47 237.25,44 | 237.88,41.88 237.25,42.5 237.25,44 | 237.25,44 193,44 188.25,48.75 188.25,49.5 J1.1 | v258,54.25 258.62,54.88 | v241.5,54.25 240.5,53.25 239.5,53.25 IC2.8
  Top 0.406: 264.25,42 264.25,46.5 263,47.75 261.5,47.75 | IC9.2 261.58,42 264.25,42 | v165,41.25 162.5,38.75 121,38.75
  Bottom 0.406: J1.1 188,49.75 186.25,51.5 184.25,51.5 182.5,49.75 J1.3 | v241.5,54.25 v258,54.25 | v165,41.25 172.75,41.25 175.5,44 177.5,44 178.5,45 182.25,45 184,46.75 J1.21

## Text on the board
Top: - 5V + | ADWin Digital Buffer Rev:F J.Thywissen Labs, University of Toronto, Physics
tNames: 1A | 0.5A
Target: ADWin Digital Buffer | J. Thywissen Labs | Stummer/Myrskog Aug'05 | F | 0.18mm | 0.36mm | 0.18mm | 0.25mm | 0.5mm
